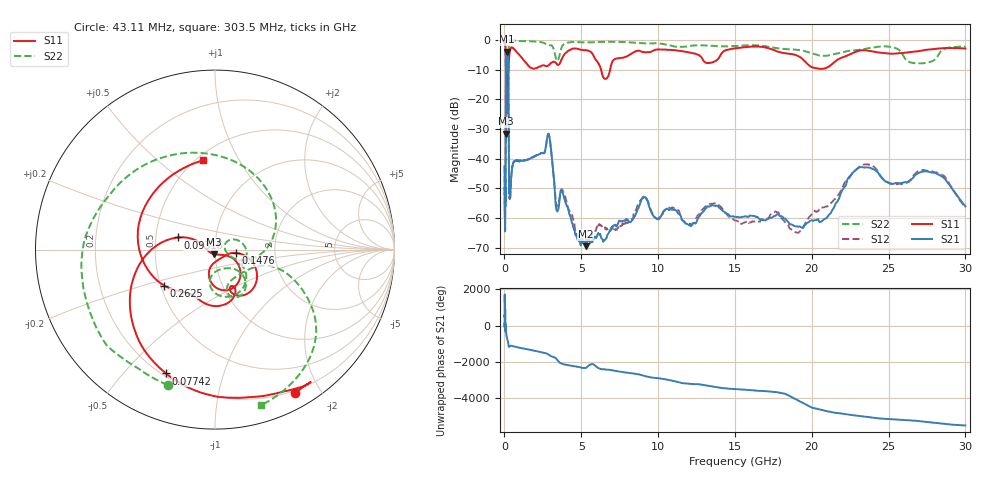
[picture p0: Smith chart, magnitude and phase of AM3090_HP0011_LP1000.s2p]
! Date/Time: Thu, Feb 28, 2019 1:56 PM
! Network Analyzer: Agilent Technologies E8364B Rev: A.07.50.67
! Sweep from 0.010 to 30.000 GHz, 1601 Points, Sweep Type: LOG
! Power Supply: 5.022 V, 0.002 A
# Hz S DB R 50
!freq MagS11 AngS11 MagS21 AngS21 MagS12 AngS12 MagS22 AngS22
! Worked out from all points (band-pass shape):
!   1601 points, 10 MHz to 30 GHz, reference 50 ohm
!   highest |S21| = -3.92 dB at 150.6 MHz (marker M1); lowest = -69.5 dB at 5.285 GHz (marker M2)
!   |S21| within 3 dB of the highest: 102.5 MHz to 239 MHz (136.5 MHz wide, 79.9 % of centre)
!   lowest |S11| = -31.6 dB at 100.9 MHz (marker M3), VSWR 1.05, Z = 49.3 - j2.52 ohm
!   |S11| at or under -10 dB: 91.52 MHz to 257.7 MHz (166.2 MHz wide, 95.2 % of centre); 6.289 GHz to 6.876 GHz (587.4 MHz wide, 8.92 % of centre)
!   |S22| runs from -25.3 to -0.1 dB; largest |S21 - S12| = 0.012
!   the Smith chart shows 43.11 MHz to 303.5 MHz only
!   S11 on the Smith chart (normalised r, x): 43.11 MHz: 0.17, -1.70; 77.42 MHz: 0.21, -0.66; 93.16 MHz: 0.65, +0.09; 147.6 MHz: 1.26, -0.05; 262.5 MHz: 0.52, -0.24; 303.5 MHz: 0.54, +0.72
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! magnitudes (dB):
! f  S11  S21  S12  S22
! 10 MHz  -0.2  -42.5  -43.0  -0.6
! 38.04 MHz  -0.5  -60.3  -60.5  -1.5
! 43.11 MHz  -0.8  -64.2  -62.1  -1.9
! 48.37 MHz  -0.8  -50.8  -47.4  -1.9
! 77.42 MHz  -2.6  -45.8  -46.4  -4.8
! 93.16 MHz  -13.3  -14.3  -14.3  -12.0
! 100.9 MHz  -31.6  -7.5  -7.5  -24.5
! 116.7 MHz  -12.7  -5.0  -5.0  -16.7
! 144.7 MHz  -22.2  -3.9  -3.9  -16.3
! 147.6 MHz  -18.7  -3.9  -3.9  -15.9
! 150.6 MHz  -16.0  -3.9  -3.9  -15.2
! 262.5 MHz  -9.2  -16.4  -16.4  -8.8
! 303.5 MHz  -6.0  -51.2  -50.9  -0.9
! 550.5 MHz  -2.7  -41.9  -41.8  -0.2
! 2.084 GHz  -9.5  -38.9  -38.9  -0.5
! 2.884 GHz  -8.4  -31.8  -31.7  -1.8
! 3.402 GHz  -8.0  -57.5  -56.0  -6.9
! 5.285 GHz  -3.4  -69.5  -68.2  -0.8
! 7.926 GHz  -5.6  -60.4  -61.5  -0.7
! 19.03 GHz  -5.2  -62.9  -65.0  -3.3
! 23.48 GHz  -3.4  -43.0  -41.9  -3.0
! 30 GHz  -2.8  -56.1  -56.5  -2.2
